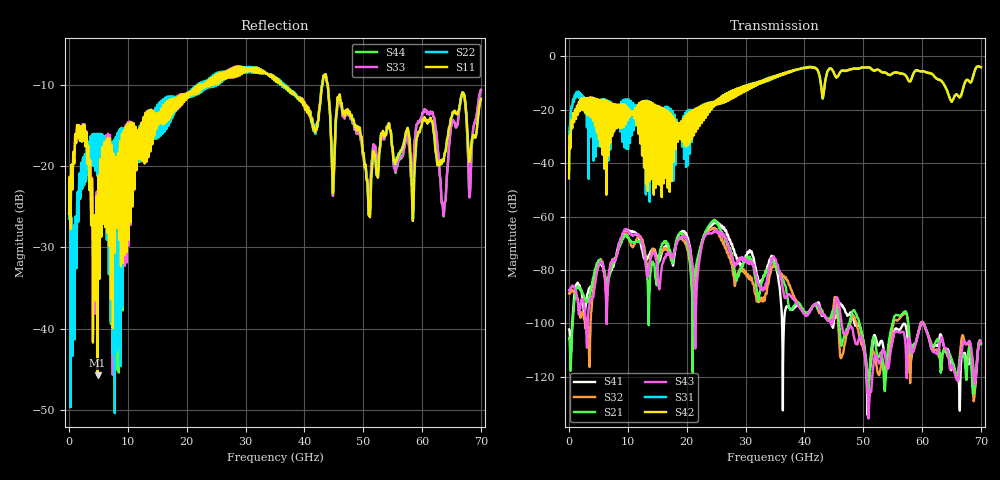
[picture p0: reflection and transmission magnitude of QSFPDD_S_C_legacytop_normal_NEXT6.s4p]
! AWR Design Environment (8415) Thu Dec 20 13:55:32 2018
! Document = 'CHANNEL TEST'
! nPorts: 4, nXvals: 7001
# HZ S DB R 50
!Freq DBS11 AngS11 DBS12 AngS12 DBS13 AngS13 DBS14 AngS14
!	DBS21 AngS21 DBS22 AngS22 DBS23 AngS23 DBS24 AngS24
!	DBS31 AngS31 DBS32 AngS32 DBS33 AngS33 DBS34 AngS34
!	DBS41 AngS41 DBS42 AngS42 DBS43 AngS43 DBS44 AngS44
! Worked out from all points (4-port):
!   7000 points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, 10 MHz to 70 GHz, reference 50 ohm
!   strongest paths, dB at 10 MHz, 17.51 GHz, 35.01 GHz, 52.51 GHz, 70 GHz:
!     S42: -45.6, -25.5, -7.4, -5.0, -4.0
!     S31: -42.3, -24.0, -7.5, -5.0, -4.0
!     S43: -87.6, -75.0, -75.9, -113.7, -107.0
!     S21: -105.5, -76.8, -78.1, -112.7, -107.8
!     S32: -88.8, -76.1, -78.9, -118.7, -107.5
!     S41: -102.3, -76.5, -77.1, -108.2, -107.2
!   lowest |S11| = -45.7 dB at 4.85 GHz (marker M1), VSWR 1.01, Z = 49.9 + j0.506 ohm
!   |S11| at or under -10 dB: start of sweep to 22.11 GHz; 36.16 GHz to 43.05 GHz (6.896 GHz wide, 17.4 % of centre); 43.97 GHz to end of sweep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
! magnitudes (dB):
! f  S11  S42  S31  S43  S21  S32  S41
! 10 MHz  -25.9  -45.6  -42.3  -87.6  -105.5  -88.8  -102.3
! 1.28 GHz  -16.1  -19.3  -13.3  -89.2  -86.9  -89.7  -85.3
! 4.85 GHz  -45.7  -16.7  -20.5  -79.8  -77.3  -78.1  -79.1
! 21.13 GHz  -10.6  -21.7  -24.3  -83.6  -89.1  -93.2  -86.4
! 25.01 GHz  -10.0  -17.1  -17.2  -65.1  -61.6  -64.5  -61.8
! 28.46 GHz  -8.2  -12.8  -13.0  -77.8  -83.7  -83.9  -75.4
! 70 GHz  -11.8  -4.0  -4.0  -107.0  -107.8  -107.5  -107.2
